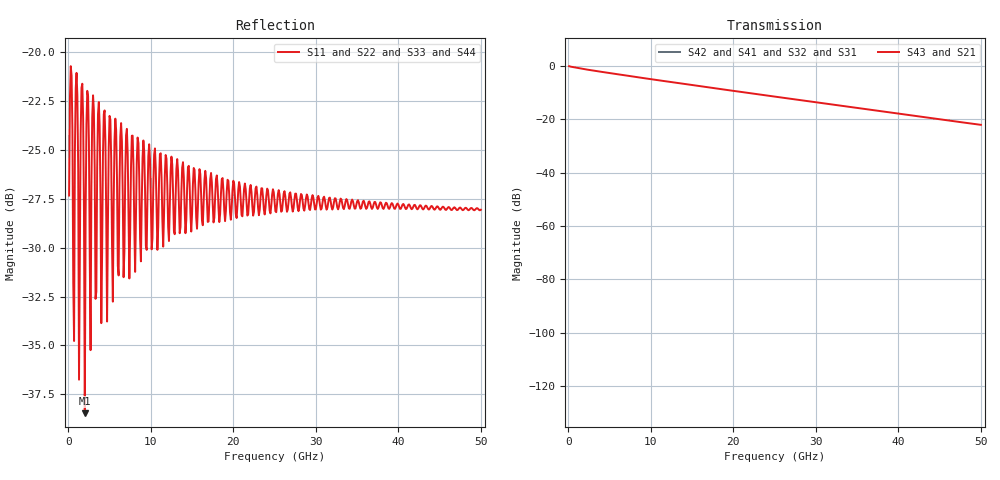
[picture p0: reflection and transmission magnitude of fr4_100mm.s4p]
! Touchstone Ver. 1.0
! Number of ports is 4
! port1 ->  port2
! port3 ->  port4
! Touchstone Ver. 1.0
! Number of ports is 4
# Hz	S	RI	R	50.000000
! SCATTERING PARAMETERS  :
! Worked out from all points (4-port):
!   500 points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, 100 MHz to 50 GHz, reference 50 ohm
!   strongest paths, dB at 100 MHz, 12.6 GHz, 25.1 GHz, 37.6 GHz, 50 GHz:
!     S43: -0.2, -6.2, -11.6, -16.9, -22.1
!     S21: -0.2, -6.2, -11.6, -16.9, -22.1
!     S42: -, -, -, -, -
!     S41: -, -, -, -, -
!     S32: -, -, -, -, -
!     S31: -, -, -, -, -
!   lowest |S11| = -38.5 dB at 2 GHz (marker M1), VSWR 1.02, Z = 48.8 + j0.074 ohm
!   |S11| at or under -10 dB: start of sweep to end of sweep
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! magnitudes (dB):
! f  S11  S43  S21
! 100 MHz  -27.3  -0.2  -0.2
! 1.7 GHz  -21.6  -1.1  -1.1
! 2 GHz  -38.5  -1.3  -1.3
! 2.3 GHz  -22.0  -1.4  -1.4
! 2.7 GHz  -35.2  -1.6  -1.6
! 3 GHz  -22.2  -1.8  -1.8
! 50 GHz  -28.1  -22.1  -22.1
